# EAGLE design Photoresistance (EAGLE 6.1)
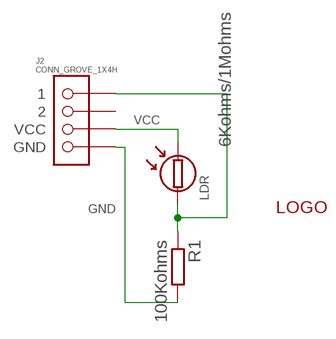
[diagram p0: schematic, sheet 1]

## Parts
J2  CONN_GROVE_1X4H  [GROVE_90_1X4]
LDR  6Kohms/1Mohms  LDRREF-PP-17460003  [NORPS-12]
R1  100Kohms  R-EU_R0603  [R0603]
U$5  LOGOSERIGRAPHIE  [LOGOSERIGRAPHIE]

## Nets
GND: J2.1(GND) R1.2
N$5: J2.4 LDR.P$1 R1.1
VCC: J2.2(VCC) LDR.P$2
Unconnected: J2.3

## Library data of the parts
J2 = boulo:CONN_GROVE_1X4
LDR = boulo:LDR
R1 = rcl:R-EU_: RESISTOR, European symbol
U$5 = boulo:LOGO

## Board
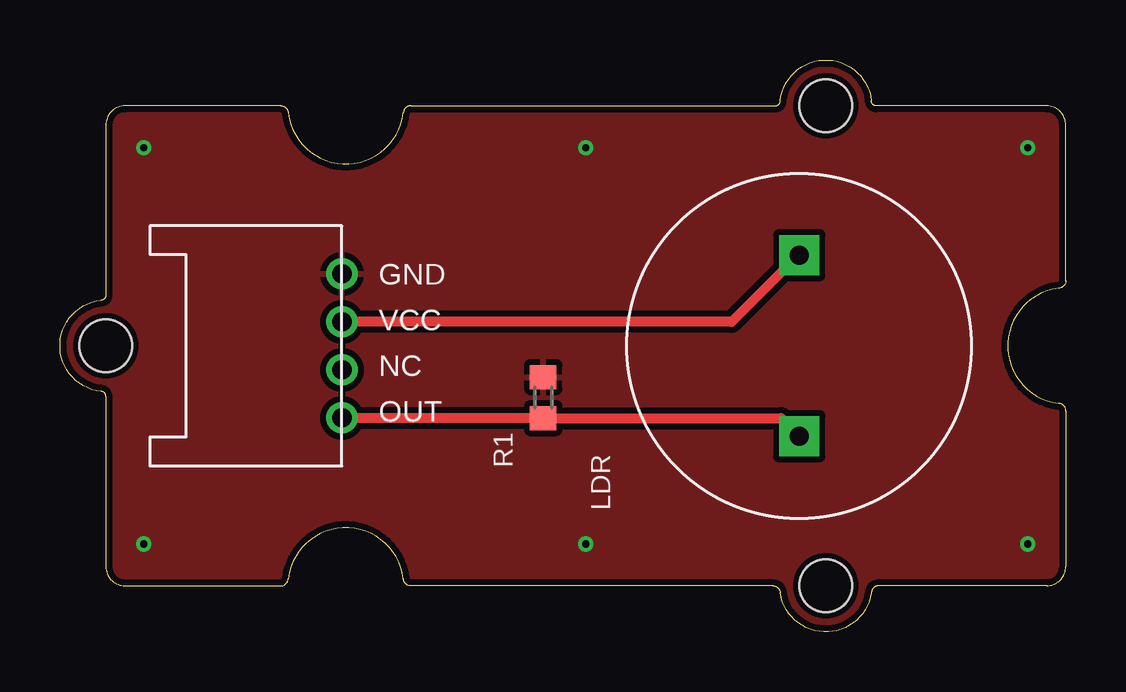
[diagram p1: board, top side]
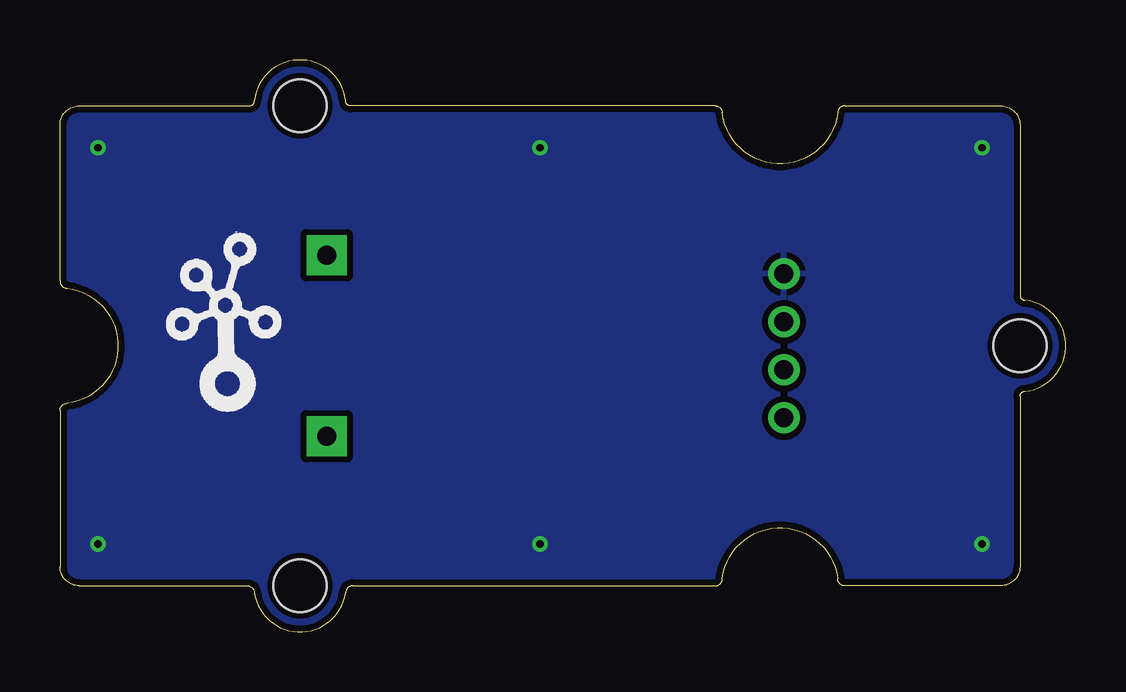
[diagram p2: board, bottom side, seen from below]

Size 41.91 x 23.83 mm. Coordinates in mm from the lower left corner, seen from the top.
Copper layers (1*16): Top 0.035mm / dielectric 1.5mm / Bottom 0.035mm
Design rules: minimum track width 6mil, minimum drill 12mil, track to track 6mil, track to pad 6mil, pad to pad 6mil, via to via 6mil, smd to smd 0mil, copper to edge 10mil, drill to drill 10mil, minimum pad ring 10mil, minimum via ring 6mil, stop-mask expansion 2mil, vias tented up to drill 25mil, thermal gap 10mil

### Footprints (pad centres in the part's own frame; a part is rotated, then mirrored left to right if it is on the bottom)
GROVE_90_1X4 = drill 0.8: 1 0,3; 2 0,1; 3 0,-1; 4 0,-3
NORPS-12 = drill 0.8 pad 1.676 square: P$1 -3.77,0; P$2 3.77,0
R0603 = smd 1 x 1.1: 1 -0.85,0; 2 0.85,0
2U-DIM-W/DRILL = hole 2.2: -10,-10; -10,10; 20,0

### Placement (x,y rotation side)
J2  11.75,11.92 0 top
LDR  30.8,11.92 90 top
R1  20.13,9.76 90 top
U$2  [2U-DIM-W/DRILL]  21.91,11.92 180 top
U$4  [TWIGLOGO]  34.99,10.14 0 bottom
U$5  21.4,11.54 0 bottom

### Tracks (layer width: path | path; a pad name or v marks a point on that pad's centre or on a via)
GND  (via drill 0.3 pad 0.64)
  other vias: 3.49,3.67 21.91,3.67 21.91,20.18 40.32,3.67 40.32,20.18 3.49,20.18
  pour Top (isolate 0.254): 42.23,-0.14 -0.32,-0.14 -0.32,23.99 42.23,23.99
  pour Bottom (isolate 0.254): 42.23,-0.14 -0.32,-0.14 -0.32,23.99 42.23,23.99
N$5
  Top 0.406: LDR.P$1 30.04,8.91 R1.1 J2.4 11.75,8.87 J2.4
VCC
  Top 0.406: LDR.P$2 30.8,15.73 27.99,12.92 J2.2

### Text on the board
tPlace: GND | VCC | NC | OUT
Reference: Photoresistance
